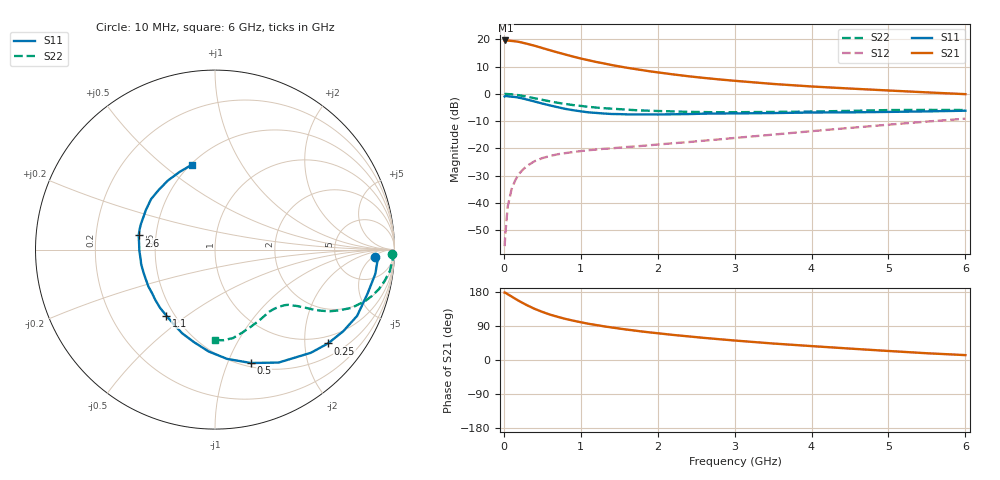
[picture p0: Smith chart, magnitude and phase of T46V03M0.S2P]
! Infineon Technologies  Discrete & RF Semiconductors
! BFR182T
! Si NPN RF Bipolar Junction Transistor in SC75
! VCE = 6 V  IC = 3 mA
! Common Emitter S-Parameters:  October  1999
# GHz  S  MA  R  50
!  f  S11  S21  S12  S22
! GHz  MAG  ANG  MAG  ANG  MAG  ANG  MAG  ANG
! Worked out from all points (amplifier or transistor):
!   36 points, 10 MHz to 6 GHz, reference 50 ohm
!   highest |S21| = 19.6 dB at 20 MHz (marker M1)
!   |S21| within 3 dB of that: start of sweep to 527.3 MHz
!   unconditionally stable (mu >= 1): 1.774 GHz to 4.252 GHz
!   at 250 MHz: K = 0.19, MSG = 23.2 dB, |S12| = -27.8 dB
!   at 1.4 GHz: K = 0.88, MSG = 15.3 dB, |S12| = -20.0 dB
!   at 6 GHz: K = 0.84, MSG = 4.5 dB, |S12| = -9.1 dB
!   lowest NFmin = 1.10 dB at 450 MHz
!   S11 on the Smith chart (normalised r, x): 10 MHz: 15, -6; 250 MHz: 0.80, -2.55; 500 MHz: 0.54, -1.22; 1.1 GHz: 0.45, -0.42; 2.6 GHz: 0.40, +0.08; 6 GHz: 0.51, +0.63
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0.01  0.8947 -2.7  9.477 177.9  0.0016 77.2  0.9868 -1.4
0.02  0.9103 -2.2  9.536 177.6  0.0027 87.7  0.9984 -1.5
0.05  0.9035 -8.6  9.49 173.6  0.0085 88.5  0.9898 -3.6
0.1  0.8843 -16.3  9.343 167.7  0.0177 81.4  0.9811 -7.1
0.15  0.8736 -25.0  9.18 161.4  0.0262 76.3  0.9611 -10.4
0.2  0.847 -32.5  8.955 155.5  0.0344 73.6  0.94 -13.5
0.25  0.8184 -39.7  8.624 150.0  0.0409 68.9  0.9131 -16.3
0.3  0.7847 -47.1  8.295 144.7  0.0475 66.4  0.8869 -18.7
0.4  0.7224 -60.6  7.622 135.0  0.058 60.3  0.8287 -23.0
0.5  0.6629 -72.4  6.928 127.0  0.0661 55.7  0.7757 -25.8
0.6  0.6126 -83.7  6.302 119.8  0.0723 53.3  0.7273 -28.2
0.8  0.529 -102.7  5.264 108.5  0.0816 48.5  0.6517 -31.1
0.9  0.5009 -111.4  4.825 103.9  0.0854 47.7  0.6213 -32.0
1.1  0.4568 -126.5  4.136 95.6  0.0923 46.6  0.5782 -33.6
1.3  0.435 -139.8  3.614 88.9  0.098 46.8  0.545 -35.0
1.6  0.4196 -156.6  3.009 80.2  0.1058 47.9  0.5116 -37.0
2.2  0.4216 -179.2  2.273 66.2  0.1238 51.9  0.4756 -42.5
2.6  0.4324 169.5  1.959 58.4  0.1382 54.3  0.4624 -46.9
3.5  0.4435 150.4  1.518 43.5  0.1783 58.2  0.4653 -57.9
4.5  0.4569 133.5  1.25 30.1  0.2369 58.5  0.4866 -71.7
5.5  0.4758 114.4  1.063 17.8  0.3095 55.6  0.5069 -84.6
6  0.4902 105.2  0.986 12.9  0.3498 52.6  0.5044 -90.3
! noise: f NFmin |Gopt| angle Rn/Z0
0.45  1.1  0.37  30  0.33
0.9  1.2  0.35  61  0.26
1.8  1.85  0.27  133  0.2
